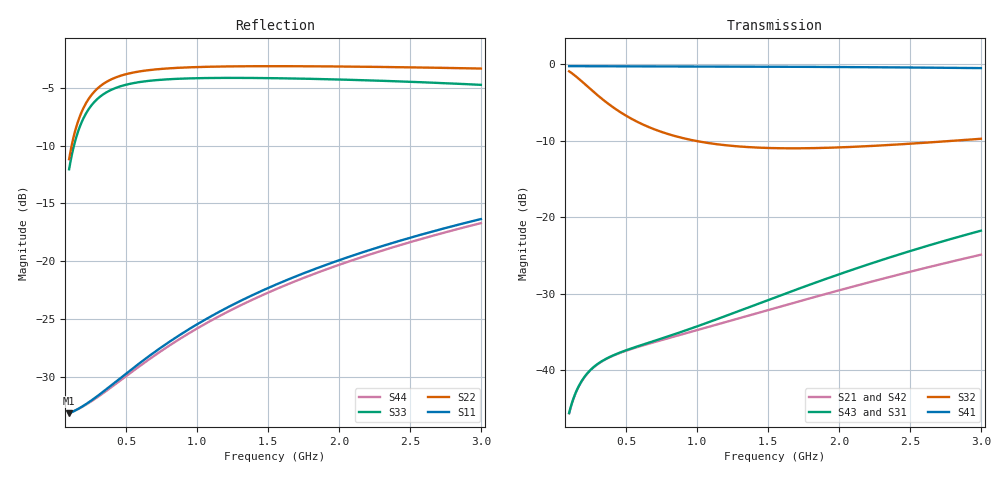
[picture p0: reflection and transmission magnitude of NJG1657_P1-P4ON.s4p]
! NJG1657MD7(1bit control high power DPDT switch) S-parameter
! VDD=2.85V, VCTL(H)=2.6V, VCTL(L)=0V
! P1-P4 ON mode
! Port1...P1, Port2...P2, Port3...P3, Port4...P4
# hz S ma R 50
! 4 Port Network Data from SP1.SP block
! freq  magS11  angS11  magS12  angS12  magS13  angS13  magS14  angS14
!  magS21  angS21  magS22  angS22  magS23  angS23  magS24  angS24
!  magS31  angS31  magS32  angS32  magS33  angS33  magS34  angS34
!  magS41  angS41  magS42  angS42  magS43  angS43  magS44  angS44
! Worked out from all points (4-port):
!   291 points, 100 MHz to 3 GHz, reference 50 ohm
!   strongest paths, dB at 100 MHz, 820 MHz, 1.55 GHz, 2.28 GHz, 3 GHz:
!     S41: -0.2, -0.3, -0.3, -0.4, -0.5
!     S32: -0.9, -9.2, -11.0, -10.6, -9.7
!     S43: -45.6, -35.4, -30.5, -25.7, -21.7
!     S31: -45.6, -35.5, -30.6, -25.9, -21.9
!     S21: -45.6, -35.7, -31.9, -28.2, -24.9
!     S42: -45.6, -35.7, -31.9, -28.3, -25.1
!   lowest |S11| = -33.2 dB at 100 MHz (marker M1), VSWR 1.04, Z = 52.2 - j0.538 ohm
!   |S11| at or under -10 dB: start of sweep to end of sweep
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1e8  0.02191 -13.6  0.005244 66.1  0.005258 67.1  0.972 -1.3
     0.005244 66.1  0.2767 -109.4  0.8997 -17.2  0.005261 66.1
     0.005258 67.1  0.8997 -17.2  0.2502 -109.7  0.005266 67.1
     0.972 -1.3  0.005261 66.1  0.005266 67.1  0.02196 -13.4
1.7e8  0.02301 -22.4  0.00793 59.7  0.007947 61.4  0.9717 -2.2
       0.00793 59.7  0.4152 -124.7  0.8013 -26.2  0.007956 59.6
       0.007947 61.4  0.8013 -26.2  0.3749 -125.7  0.007959 61.2
       0.9717 -2.2  0.007956 59.6  0.007959 61.2  0.02297 -22.1
2.8e8  0.0255 -34.7  0.01061 52.5  0.01063 55.5  0.9713 -3.7
       0.01061 52.5  0.5449 -141.0  0.6516 -34.5  0.01065 52.4
       0.01063 55.5  0.6516 -34.5  0.4914 -143.0  0.01065 55.2
       0.9713 -3.7  0.01065 52.4  0.01065 55.2  0.02524 -34.5
4.6e8  0.03109 -50.3  0.01303 48.9  0.01306 54.0  0.9707 -6.0
       0.01303 48.9  0.6355 -156.8  0.4871 -38.6  0.01307 48.7
       0.01306 54.0  0.4871 -38.6  0.5722 -160.1  0.0131 53.5
       0.9707 -6.0  0.01307 48.7  0.0131 53.5  0.03038 -50.7
7.1e8  0.04069 -65.1  0.01539 51.1  0.01561 59.6  0.9697 -9.2
       0.01539 51.1  0.6777 -168.9  0.373 -36.3  0.01542 50.8
       0.01561 59.6  0.373 -36.3  0.6086 -174.1  0.0157 58.7
       0.9697 -9.2  0.01542 50.8  0.0157 58.7  0.0393 -66.7
1.52e9  0.07737 -91.0  0.02505 64.0  0.02887 80.4  0.9645 -19.8
        0.02505 64.0  0.6999 171.7  0.2836 -22.1  0.02497 63.4
        0.02887 80.4  0.2836 -22.1  0.6211 160.6  0.02925 78.1
        0.9645 -19.8  0.02497 63.4  0.02925 78.1  0.0739 -96.6
3e9  0.1522 -118.8  0.05699 67.6  0.08012 84.1  0.9442 -39.3
     0.05699 67.6  0.6836 150.4  0.3261 -15.2  0.05563 66.2
     0.08012 84.1  0.3261 -15.2  0.5809 126.9  0.08179 79.0
     0.9442 -39.3  0.05563 66.2  0.08179 79.0  0.1462 -130.5
